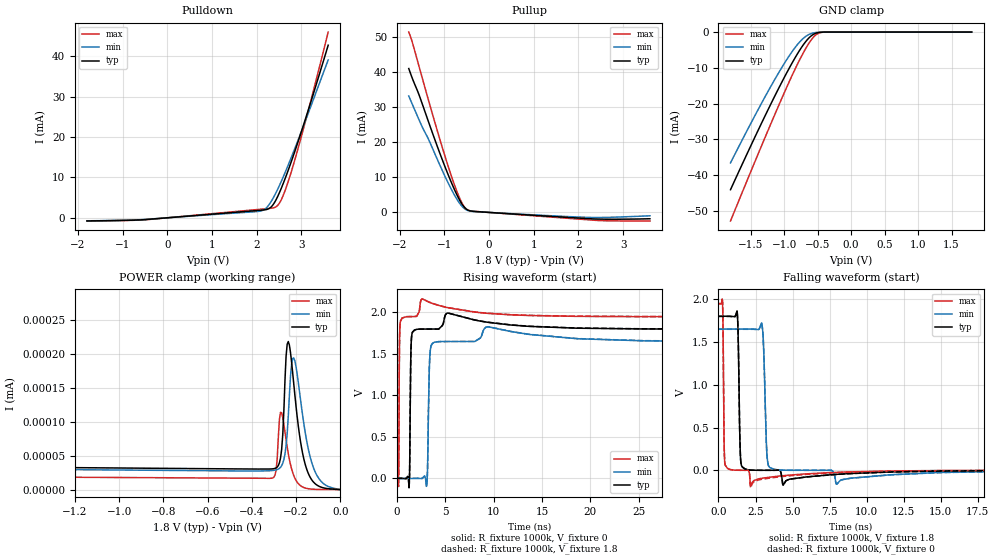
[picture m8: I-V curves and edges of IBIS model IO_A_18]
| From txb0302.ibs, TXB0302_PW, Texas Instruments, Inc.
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[Model]   IO_A_18
Model_type  3-state
Enable   Active-High
Vref =   0
Rref =   1000k
Cref =   50p
Vmeas =   0.9
| variable   typ   min   max
C_comp   3.37pF   3.16pF   3.53pF
| C_pullup   3.62pF   3.24pF   3.81pF
| C_pulldown   3.61pF   3.24pF   3.80pF
| C_tri-state   3.37pF   3.16pF   3.53pF
[Temperature Range]   40   100   -40
| Ambient temperature   25   85   -40
[Voltage range]   1.8   1.65   1.95
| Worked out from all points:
|   slope of the pulldown table from 0 to 0.27 V, typ, clamps not added: 1.1 kohm
|   slope of the pullup table from 0 to 0.27 V, typ, clamps not added: 1.21 kohm
|   GND clamp passes 1 mA (typ) near -0.59 V on its own axis
|   rising waveform, R_fixture 1000k, V_fixture 0: 20-80 % time 93.6ps typ, 150ps min, 58.5ps max; typ from 0 V to 1.8 V
|   falling waveform, R_fixture 1000k, V_fixture 1.8: 20-80 % time 102ps typ, 159ps min, 62.3ps max; typ from 1.8 V to 0.002 V
|   rising waveform, R_fixture 1000k, V_fixture 1.8: 20-80 % time 93.8ps typ, 151ps min, 58.6ps max; typ from 0.002 V to 1.8 V
|   falling waveform, R_fixture 1000k, V_fixture 0: 20-80 % time 102ps typ, 159ps min, 62.4ps max; typ from 1.8 V to 0 V
[GND Clamp]
| IO_A_18
|   Voltage   I(typ)   I(min)   I(max)
-1.8V     -44.03mA   -36.54mA   -52.78mA
-1.53V    -33.08mA   -26.69mA   -40.45mA
-1.295V   -23.82mA   -18.44mA   -29.91mA
-1.1V     -16.42mA   -11.97mA   -21.34mA
-940mV    -10.66mA   -7.1mA     -14.54mA
-815mV    -6.519mA   -3.818mA   -9.525mA
-715mV    -3.614mA   -1.788mA   -5.862mA
-615mV    -1.392mA   -570.2uA   -2.718mA
-525mV    -328.4uA   -135.8uA   -785.2uA
-460mV    -77.79uA   -34.89uA   -182.9uA
-365mV    -6.097uA   -3.221uA   -9.086uA
1.8V      303.3pA    68.73nA    29.48pA
[POWER Clamp]
| IO_A_18
|   Voltage   I(typ)   I(min)   I(max)
-1.8V     249.5nA    33.48nA    134.8uA
-1.78V    136.7nA    32.29nA    68.41uA
-1.755V   74.54nA    31.51nA    24.38uA
-1.665V   35.01nA    30.68nA    329.2nA
-1.63V    33.86nA    30.55nA    73.17nA
-1.575V   33.36nA    30.37nA    22.16nA
-295mV    31.28nA    28.68nA    21.38nA
-270mV    46.7nA     32.91nA    114nA
-235mV    218.3nA    108.2nA    53.04nA
-210mV    155.1nA    194nA      20.51nA
-150mV    28.48nA    68.73nA    1.64nA
0V        0A         0A         0A
[Pulldown]
| IO_A_18
|   Voltage   I(typ)   I(min)   I(max)
-1.8V     -774.1uA   -745uA     -797.4uA
-510mV    -457.1uA   -406.1uA   -507.9uA
2.055V    1.834mA    1.613mA    2.09mA
2.18V     1.972mA    2.139mA    2.217mA
2.29V     2.387mA    3.475mA    2.331mA
2.365V    3.231mA    4.824mA    2.447mA
2.445V    4.73mA     6.524mA    2.825mA
2.52V     6.525mA    8.286mA    3.85mA
2.6V      8.689mA    10.29mA    5.736mA
2.82V     15.38mA    16.24mA    13.1mA
3.15V     26.53mA    25.79mA    26.39mA
3.6V      42.75mA    39.09mA    46.02mA
[Pullup]
| IO_A_18
|   Voltage   I(typ)   I(min)   I(max)
-1.8V     40.91mA    33.09mA    51.29mA
-1.72V    38.11mA    30.74mA    48.35mA
-1.565V   33.27mA    26.2mA     41.29mA
-1.235V   21.37mA    17.25mA    26.45mA
-895mV    10.01mA    7.789mA    12.24mA
-770mV    6.311mA    4.781mA    7.6mA
-665mV    3.589mA    2.658mA    4.199mA
-580mV    1.854mA    1.379mA    2.056mA
-505mV    883.4uA    695.4uA    912.4uA
-315mV    266.9uA    233.2uA    303.4uA
2.185V    -1.741mA   -1.399mA   -2.062mA
3.6V      -1.802mA   -955.9uA   -2.439mA
[Ramp]
| IO_A_18
| variable   typ   min   max
dV/dt_r   1.27/1.35E-10   1.15/2.13E-10   1.36/8.12E-11
dV/dt_f   1.22/1.30E-10   1.13/2.10E-10   1.31/8.10E-11
R_load = 1000k
[Rising Waveform]
| IO_A_18
R_fixture =   1000k
C_fixture =   0
L_fixture =   0
V_fixture =   0
V_fixture_min = 0
V_fixture_max = 0
|   Time   V(typ)   V(min)   V(max)
0s        427.9nV    2.161uV    53.72nV
189ps     367.4nV    2.161uV    -96.45mV
365ps     4.644uV    2.16uV     1.878V
1.277ns   -113.1mV   2.067uV    1.949V
1.533ns   1.705V     7.658uV    1.95V
2.621ns   1.799V     -1.227mV   2.163V
3.117ns   1.8V       -56.38mV   2.136V
3.413ns   1.8V       1.456V     2.12V
3.885ns   1.8V       1.64V      2.101V
37.16ns   1.798V     1.649V     1.948V
[Falling Waveform]
| IO_A_18
R_fixture =   1000k
C_fixture =   0
L_fixture =   0
V_fixture =   1.8
V_fixture_min = 1.65
V_fixture_max = 1.95
|   Time   V(typ)   V(min)   V(max)
0s        1.8V       1.65V      1.95V
277ps     1.8V       1.65V      1.963V
429ps     1.8V       1.65V      83.16mV
1.261ns   1.859V     1.65V      960.1uV
1.501ns   112.5mV    1.65V      452.3uV
2.173ns   2.772mV    1.65V      -185.2mV
2.941ns   294.9uV    1.698V     -92.93mV
3.277ns   195.9uV    168.5mV    -84.56mV
3.725ns   133.8uV    11.63mV    -74.85mV
37.16ns   1.961mV    2.05mV     1.902mV
[Rising Waveform]
| IO_A_18
R_fixture =   1000k
C_fixture =   0
L_fixture =   0
V_fixture =   1.8
V_fixture_min = 1.65
V_fixture_max = 1.95
|   Time   V(typ)   V(min)   V(max)
0s        1.98mV     2.064mV    1.901mV
189ps     1.98mV     2.064mV    -94.58mV
373ps     1.984mV    2.064mV    1.885V
1.277ns   -111.1mV   2.064mV    1.949V
1.533ns   1.705V     2.07mV     1.95V
2.621ns   1.799V     835.1uV    2.163V
3.117ns   1.8V       -54.3mV    2.136V
3.413ns   1.8V       1.457V     2.121V
3.885ns   1.8V       1.64V      2.101V
37.16ns   1.8V       1.651V     1.95V
[Falling Waveform]
| IO_A_18
R_fixture =   1000k
C_fixture =   0
L_fixture =   0
V_fixture =   0
V_fixture_min = 0
V_fixture_max = 0
|   Time   V(typ)   V(min)   V(max)
0s        1.798V     1.648V     1.948V
277ps     1.798V     1.648V     1.961V
429ps     1.798V     1.648V     82.99mV
1.261ns   1.857V     1.648V     920.9uV
1.501ns   112.2mV    1.648V     413.1uV
2.181ns   2.642mV    1.648V     -204.9mV
2.941ns   254.7uV    1.695V     -104.4mV
3.277ns   155.9uV    167.9mV    -95.2mV
3.725ns   93.88uV    11.59mV    -84.54mV
37.16ns   -17.07uV   -5.21uV    -782nV
